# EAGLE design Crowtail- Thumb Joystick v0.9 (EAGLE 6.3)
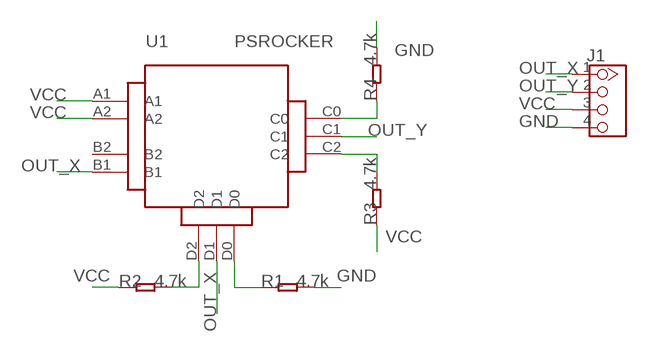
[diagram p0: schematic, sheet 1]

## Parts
J1  TWIG-2.0-LEADED  [4P-LEADED-2.0]
R1  4.7k  R-0603  [0603]
R2  4.7k  R-0603  [0603]
R3  4.7k  R-0603  [0603]
R4  4.7k  R-0603  [0603]
U1  PSROCKER  [PSROCKER]

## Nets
GND: J1.4 R1.2 R4.2
N$3: R3.2 U1.C2
N$4: R2.2 U1.D2
N$5: R1.1 U1.D0
N$6: R4.1 U1.C0
OUT_X: J1.1 U1.B1 U1.D1
OUT_Y: J1.2 U1.C1
VCC: J1.3 R2.1 R3.1 U1.A1 U1.A2
Unconnected: U1.B2

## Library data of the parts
J1 = Connector:TWIG-2.0-LEADED
R1-R4 = Discrete:R*
U1 = AnlogDevice:PSROCKER

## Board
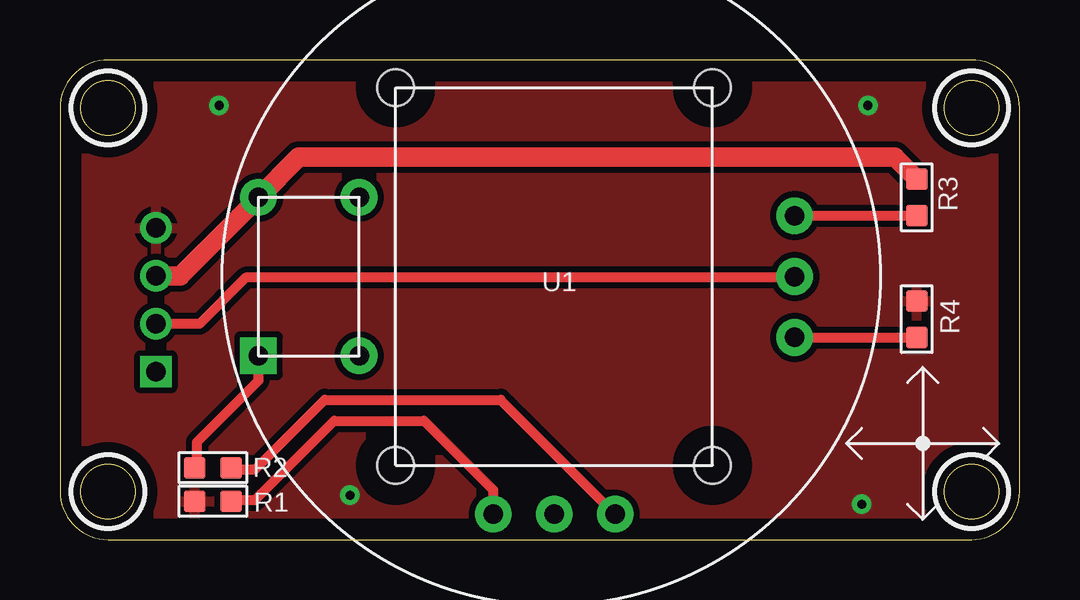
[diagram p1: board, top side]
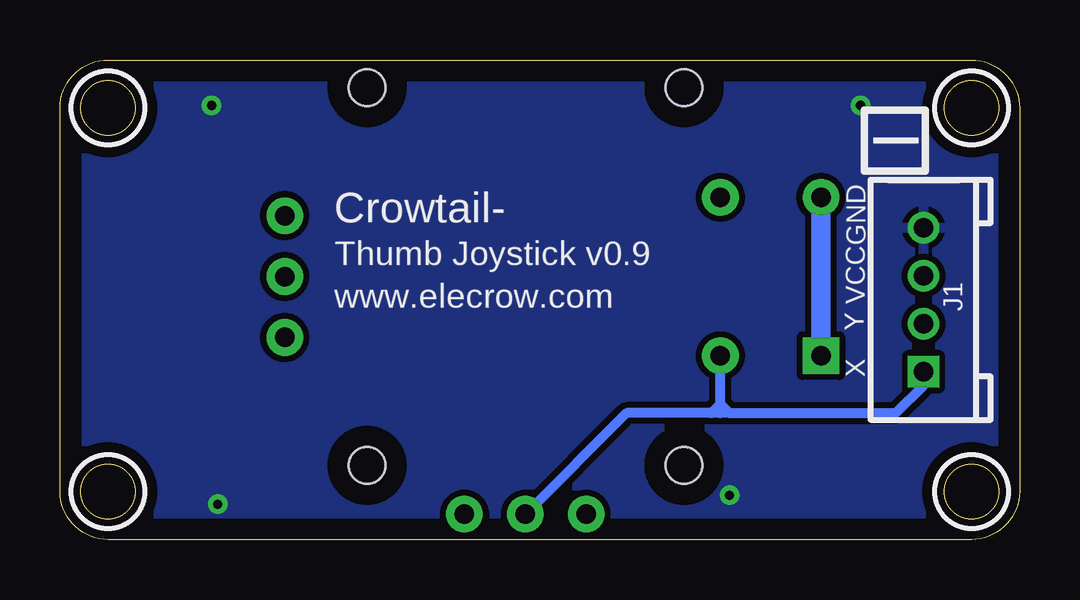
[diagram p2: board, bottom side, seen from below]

Size 40 x 20 mm. Coordinates in mm from the lower left corner, seen from the top.
Outline: 0,18 0,2 arc90 2,0 38,0 arc90 40,2 40,18 arc90 38,20 2,20 arc90 0,18
Outline: circle at 2,18 radius 1.14
Outline: circle at 2,2 radius 1.14
Outline: circle at 38,18 radius 1.14
Outline: circle at 38,2 radius 1.14
Copper layers (1*16): Top 0.035mm / dielectric 1.5mm / Bottom 0.035mm
Design rules "SeeedStudio_rule_090524 *": minimum track width 0.0025mm, minimum drill 10mil, track to track 6mil, track to pad 6mil, pad to pad 6mil, via to via 6mil, smd to smd 6mil, copper to edge 35mil, drill to drill 8mil, minimum pad ring 10mil, minimum via ring 6mil, stop-mask expansion 2mil, vias tented up to drill 100mil, thermal gap 10mil
tRestrict: area 0.5,16.5 to 3.5,19.5; area 0.5,0.5 to 3.5,3.5; area 36.5,16.5 to 39.5,19.5; area 36.5,0.5 to 39.5,3.5
bRestrict: area 0.5,16.5 to 3.5,19.5; area 0.5,0.5 to 3.5,3.5; area 36.5,16.5 to 39.5,19.5; area 36.5,0.5 to 39.5,3.5

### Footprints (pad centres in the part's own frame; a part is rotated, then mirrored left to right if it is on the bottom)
4P-LEADED-2.0 = drill 0.8 pad 1.27 square: 1 -3,0 | drill 0.8 pad 1.27: 2 -1,0; 3 1,0; 4 3,0
0603 = smd 0.889 x 0.889: 1 -0.762,0; 2 0.762,0
PSROCKER = drill 0.813 pad 1.524 square: A1 -3.302,12.319 | drill 0.813 pad 1.524: A2 3.302,12.319; B1 -3.302,8.128; B2 3.302,8.128; C0 -2.54,-10.033; C1 0,-10.033; C2 2.54,-10.033; D0 -9.906,2.54; D1 -9.906,0; D2 -9.906,-2.54 | hole 1.524: -7.874,6.604; 7.874,6.604; 7.874,-6.604; -7.874,-6.604

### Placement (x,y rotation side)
J1  4,10 90 bottom
R1  6.37,1.6 180 top
R2  6.37,2.99 0 top
R3  35.71,14.27 270 top
R4  35.71,9.19 90 top
U1  20.6,10.97 90 top

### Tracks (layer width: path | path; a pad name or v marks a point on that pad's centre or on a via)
GND  (via drill 0.38 pad 0.81)
  other vias: 6.63,18.11 33.42,1.47 33.68,18.11 12.09,1.85
  pour Bottom (isolate 0.254): -0.62,-0.32 -0.49,20.77 40.53,20.51 40.4,-0.57
  pour Top (isolate 0.254): -0.62,-0.32 -0.49,20.77 40.4,20.51 40.27,-0.57
N$3
  Top 0.406: U1.C2 R3.2
N$4
  Top 0.406: R2.2 7.21,2.92 8.13,2.92 11.04,5.83 18.37,5.83 U1.D2
N$5
  Top 0.406: U1.D0 18.06,2.07 15.17,4.96 11.43,4.96 8.13,1.65 7.19,1.65 R1.1
N$6
  Top 0.406: U1.C0 R4.1
OUT_X
  Bottom 0.406: 12.09,5.28 12.47,5.28 | 12.47,5.28 12.85,5.28 | 12.85,5.28 16.38,5.28 U1.D1 | 12.47,5.28 12.47,5.66 | 12.47,5.66 U1.B1 | 12.47,5.66 12.85,5.28 | 12.09,5.28 12.47,5.66 | 12.09,5.28 5.15,5.28 4,6.43 J1.1
OUT_Y
  Top 0.406: U1.C1 30.59,10.92 7.74,10.92 5.82,9 J1.2
VCC
  Top 0.406: R2.1 5.71,3.09 5.71,4.06 8.28,6.63 U1.A1
  Top 0.813: R3.1 34.8,15.95 9.96,15.95 U1.A2 5.01,11 J1.3
  Bottom 0.813: U1.A1 U1.A2

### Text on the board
bPlace: I | Crowtail- | GND | Thumb Joystick v0.9 | VCC | www.elecrow.com | Y | X
tNames: U1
